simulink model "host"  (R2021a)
settings: Solver=VariableStepAuto  StartTime=0.0  StopTime=inf  RelTol=1e-3
undefined symbols (not defined in the file): COM
libraries: c2000scilib x3

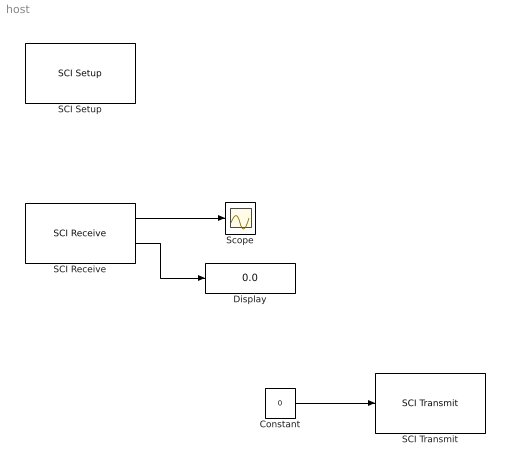
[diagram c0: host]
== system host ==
  Constant : Constant  Value=0  OutDataTypeStr=single  SampleTime=0.1
  Display : Display
  SCI Receive : c2000scilib/SCI Receive  module=COM 4  dataHead='S'  dataTail='E'  dataType=single  dataDim=2  initValue=0  errOption=Output the last received value  errValue=0  sampleTime=0.1  outputStatus=on
  SCI Setup : c2000scilib/SCI Setup  Priority=-99  commModeA=raw data  baudRateA=115200  charLenA=8  stopBitA=1  parityA=none  timeoutA=1.0  commModeB=raw data  baudRateB=115200  charLenB=8  stopBitB=1  parityB=none  timeoutB=1.0  commModeC=raw data  baudRateC=115200  charLenC=8  stopBitC=1  parityC=none  timeoutC=1.0  commModeD=raw data  baudRateD=115200  charLenD=8  stopBitD=1  parityD=none  timeoutD=1.0
  SCI Transmit : c2000scilib/SCI Transmit  module=COM 4  header='S'  tail='E'
  Scope : Scope
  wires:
  SCI Receive/1 -> Scope/1
  SCI Receive/2 -> Display/1
  Constant/1 -> SCI Transmit/1
